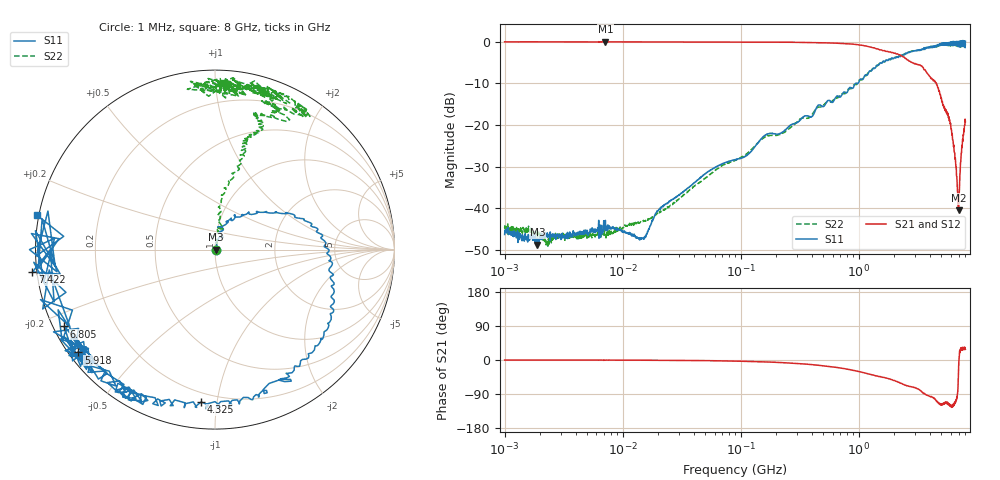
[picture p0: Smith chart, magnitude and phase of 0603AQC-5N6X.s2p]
!s-Parameter Generated by FASTRON Sdn. Bhd.
!FASTRON P/N : 0603AQC-5N6X
!Keysight Technologies: E5071C_MY46733604_B.14.02
!Date: Thu Jun 25 13:49:12 2026
!Version  :Rev00  Thu Jun 25 13:49:12 2026
!Data & Calibration Information:
!Freq  S11:SOLT2(ON)  S21:SOLT2(ON)  S12:SOLT2(ON)  S22:SOLT2(ON)
!PortZ  Port1:50+j0  Port2:50+j0
!When reading reference impedance value at option line is always used.
! Remarks : This data is being provided solely for informational purposes.
# Hz S dB R 50
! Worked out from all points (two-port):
!   1601 points, 1 MHz to 8 GHz, reference 50 ohm
!   highest |S21| = 0.02 dB at 7.138 MHz (marker M1); lowest = -40.5 dB at 6.998 GHz (marker M2)
!   |S21| within 3 dB of the highest: start of sweep to 2.145 GHz
!   lowest |S11| = -48.7 dB at 1.897 MHz (marker M3), VSWR 1.01, Z = 50.4 + j0.0274 ohm
!   |S11| at or under -10 dB: start of sweep to 940.5 MHz; 957.3 MHz to 985.4 MHz (28.08 MHz wide, 2.89 % of centre)
!   |S22| runs from -49.1 to -0.3 dB; largest |S21 - S12| = 0.015
!   S11 on the Smith chart (normalised r, x): 1 MHz: 1.01, -0.00; 4.325 GHz: 0.15, -0.90; 5.918 GHz: 0.03, -0.33; 6.805 GHz: 0.03, -0.24; 7.422 GHz: -0.01, -0.06; 8 GHz: -0.01, +0.10
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1000000  -46.30 -2.8  -0.04 -0.1  -0.05 -0.1  -44.70 3.3
1897122  -48.70 4.2  -0.05 -0.2  -0.06 -0.1  -46.50 4.6
2336708  -46.60 15.7  -0.06 -0.1  -0.05 -0.1  -48.10 23.1
4479405  -45.80 15.8  -0.04 -0.2  -0.05 -0.2  -46.60 21.7
7138274  -42.90 21.4  0.02 -0.5  -0.05 -0.1  -44.60 29.3
1.449233e7  -47.40 22.1  -0.05 -0.5  -0.06 -0.6  -43.20 38.9
2.00676e7  -40.50 38.4  -0.06 -0.7  -0.06 -0.7  -41.20 64.9
8.994653e7  -28.30 81.6  -0.08 -3.0  -0.08 -2.9  -28.50 71.7
4.006501e8  -18.00 80.1  -0.20 -12.2  -0.20 -12.3  -17.60 71.9
1.218072e9  -7.27 27.6  -1.23 -37.0  -1.23 -37.1  -7.27 76.4
1.7949e9  -4.31 4.8  -2.48 -49.5  -2.50 -49.7  -4.21 73.6
2.89772e9  -2.19 -39.2  -5.13 -71.8  -5.16 -71.8  -2.24 73.1
3.710194e9  -1.56 -69.9  -7.15 -91.3  -7.13 -91.5  -1.49 66.0
4.324643e9  -1.39 -95.2  -9.22 -100.0  -9.21 -101.0  -1.33 70.6
4.912472e9  -0.90 -117.0  -12.70 -117.0  -12.70 -117.0  -0.91 58.1
5.556285e9  -0.34 -124.0  -17.30 -112.0  -17.30 -113.0  -0.54 75.9
5.918038e9  -0.42 -143.0  -19.20 -122.0  -19.20 -123.0  -0.86 67.1
6.380696e9  -0.97 -142.0  -24.80 -116.0  -24.80 -116.0  -0.77 80.6
6.804799e9  -0.51 -153.0  -33.70 -99.9  -33.60 -101.0  -0.89 88.9
6.997574e9  -0.57 -159.0  -40.50 -34.1  -40.50 -34.9  -1.09 88.6
7.421677e9  0.21 -173.0  -26.70 30.3  -26.70 29.4  -0.46 85.6
8e9  0.10 169.0  -19.20 28.2  -19.20 27.5  -0.66 87.0
